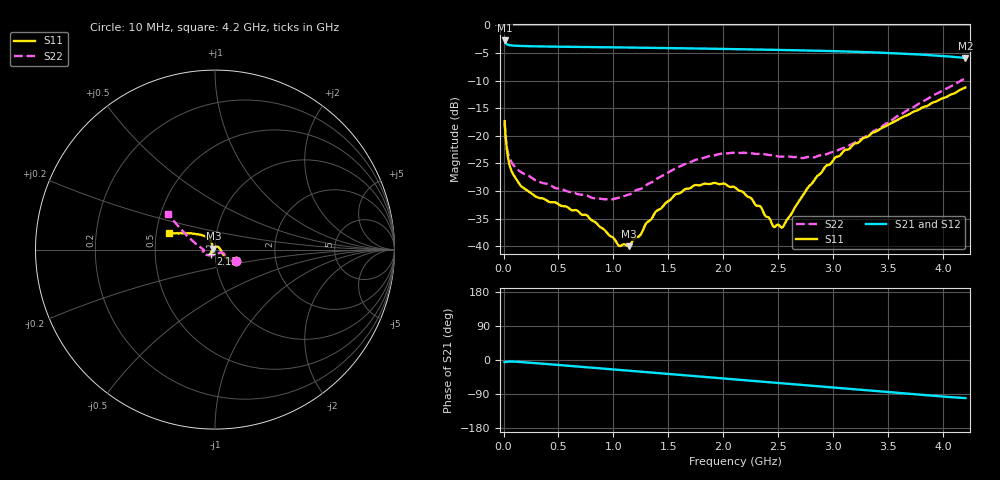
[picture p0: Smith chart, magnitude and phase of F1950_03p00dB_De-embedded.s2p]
! Integrated Device Technology
! Corporate Headquarters
! 6024 Silver Creek Valley Road
! San Jose, CA 95138  USA
! Phone:  1-408-284-8200
! Toll Free:  1-800-223-1366
! Webpage:  http://www.idt.com/
! Timing and RF Division
! 515 Groton Road, Suite 102
! Westford, MA 01886-6024
! Device:  F1950
! Description: 7-bit 0.25 dB Digital Step Attenuator
! Frequency:  150.0 -  4000.00 MHz
! Package:  4x4 mm Thin QFN Plastic Package: 24 pin
! Ports:  2 RF, 12 DC
!  Pin  1  = D0
!  Pin  2  = VDD
!  Pin  3  = Vmode
!  Pin  4  = GND
!  Pin  5  = RF1  =  Port 1
!  Pin  6  = GND
!  Pin  7  = GND
!  Pin  8  = GND
!  Pin  9  = GND
!  Pin 10  = GND
!  Pin 11  = GND
!  Pin 12  = GND
!  Pin 13  = GND
!  Pin 14  = RF2  =  Port 2
!  Pin 15  = GND
!  Pin 16  = LE
!  Pin 17  = CLK
!  Pin 18  = DATE
!  Pin 19  = D6
!  Pin 20  = D5
!  Pin 21  = D4
!  Pin 22  = D3
!  Pin 23  = D2
!  Pin 24  = D1
! State:  12
! Atten State:  3.00 dB
! Voltage:  +5.00 Volts
! Current:  Not Measured mA
! Data:  The device was measured on a the F195X evaluation board which has
!  individual transmission lines to the RF pins.  Data was collected
!  using a calibrated network analyzer.  The evaluation board was
!  de-embedded using a TRL calibration technique.
!  The reference plane is the edge of the package pin.
! Misc:  Board 2019
!  Action Tracker AT0250
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# GHz S dB R 50
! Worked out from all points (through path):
!   420 points, 10 MHz to 4.2 GHz, reference 50 ohm
!   highest |S21| = -2.75 dB at 10 MHz (marker M1); lowest = -5.9 dB at 4.2 GHz (marker M2)
!   group delay of S21, straight-line fit = 66.2 ps
!   lowest |S11| = -40.0 dB at 1.14 GHz (marker M3), VSWR 1.02, Z = 49.1 + j0.453 ohm
!   |S11| at or under -10 dB: start of sweep to end of sweep
!   |S22| runs from -31.5 to -9.6 dB; largest |S21 - S12| = 0.00079
!   S11 on the Smith chart (normalised r, x): 10 MHz: 1.26, -0.17; 2.13 GHz: 0.96, -0.05; 4.2 GHz: 0.58, +0.12
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0.01  -17.33 -28.4  -2.75 -5.6  -2.74 -5.6  -17.63 -27.7
0.04  -23.86 -35.5  -3.53 -4.3  -3.53 -4.3  -23.04 -31.7
0.06  -25.67 -31.2  -3.62 -4.0  -3.62 -4.0  -24.25 -28.0
0.16  -29.11 -13.0  -3.74 -5.4  -3.74 -5.4  -26.57 -22.6
0.3  -31.06 9.1  -3.81 -8.5  -3.81 -8.5  -28.14 -23.8
0.71  -34.24 60.1  -3.92 -18.0  -3.92 -18.1  -30.66 -41.4
0.84  -35.70 75.8  -3.95 -21.1  -3.95 -21.1  -31.28 -54.4
1.05  -39.90 120.5  -4.01 -26.1  -4.00 -26.1  -31.19 -85.1
1.14  -39.96 152.7  -4.03 -28.2  -4.03 -28.2  -30.63 -98.6
1.41  -33.37 -151.7  -4.10 -34.6  -4.10 -34.7  -27.57 -130.8
1.56  -30.65 -142.4  -4.14 -38.2  -4.14 -38.2  -25.91 -142.2
1.74  -28.93 -135.4  -4.20 -42.5  -4.19 -42.5  -24.38 -152.1
1.92  -28.51 -132.2  -4.25 -46.8  -4.25 -46.8  -23.50 -159.6
2.11  -29.39 -132.0  -4.32 -51.3  -4.32 -51.4  -23.10 -164.8
2.13  -29.75 -132.7  -4.33 -51.8  -4.33 -51.9  -23.11 -165.5
2.33  -32.69 -145.6  -4.40 -56.6  -4.40 -56.6  -23.24 -169.3
2.46  -36.51 -173.9  -4.44 -59.6  -4.44 -59.6  -23.59 -171.2
2.53  -36.61 164.4  -4.47 -61.3  -4.46 -61.3  -23.77 -173.3
2.81  -28.49 116.9  -4.58 -68.1  -4.58 -68.1  -23.89 -179.3
3.1  -22.63 120.6  -4.73 -75.3  -4.73 -75.3  -22.12 173.0
3.51  -17.86 137.8  -5.02 -85.3  -5.01 -85.3  -17.48 158.7
4.2  -11.26 160.2  -5.91 -100.5  -5.91 -100.6  -9.59 142.9
